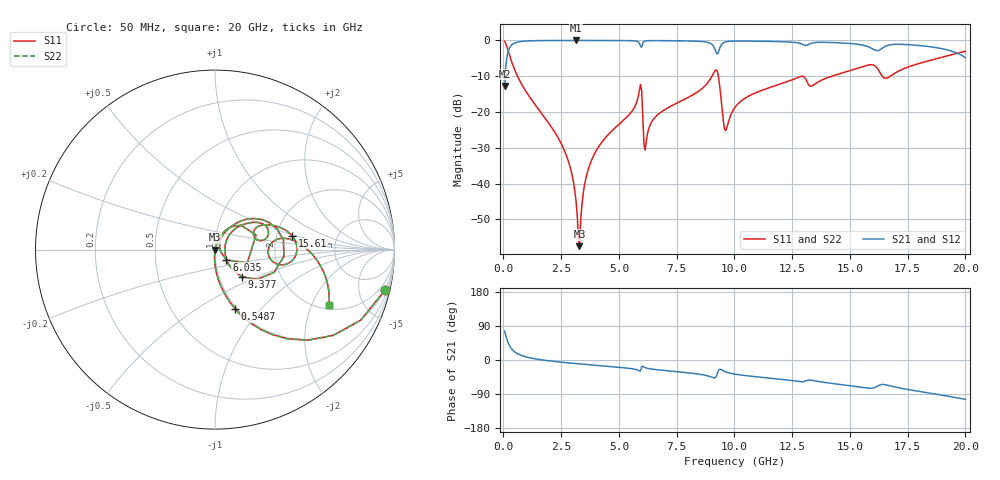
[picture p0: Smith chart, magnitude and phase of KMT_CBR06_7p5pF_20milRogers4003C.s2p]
! Data measured by Modelithics Inc. support@modelithics.com 813-866-6335
! KEMET CBR0603 7.5pF, Pad Width= 0.851mm, Pad Length= 0.64mm, Pad Gap= 0.62mm, 20mil Rogers 4003C substrate Data, January 2022
# hz S ma R 50
! 2 Port Network Data from SP1.SP block
! freq  magS11  angS11  magS21  angS21  magS12  angS12  magS22  angS22
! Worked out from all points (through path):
!   401 points, 50 MHz to 20 GHz, reference 50 ohm
!   highest |S21| = -0.01 dB at 3.142 GHz (marker M1); lowest = -12.7 dB at 50 MHz (marker M2)
!   group delay of S21, straight-line fit = 14.8 ps
!   lowest |S11| = -57.5 dB at 3.292 GHz (marker M3), VSWR 1.00, Z = 50.1 + j0.0443 ohm
!   |S11| at or under -10 dB: 610.2 MHz to 9.026 GHz (8.416 GHz wide, 175 % of centre); 9.303 GHz to 14.21 GHz (4.909 GHz wide, 41.8 % of centre); 16.4 GHz to 16.75 GHz (342.3 MHz wide, 2.07 % of centre)
!   |S22| runs from -57.5 to -0.2 dB; largest |S21 - S12| = 0
!   S11 on the Smith chart (normalised r, x): 50 MHz: 0.98, -8.32; 548.8 MHz: 0.98, -0.74; 6.035 GHz: 1.13, -0.13; 9.377 GHz: 1.28, -0.40; 15.61 GHz: 2.43, +0.47; 20 GHz: 2.21, -2.70
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5e7  0.9728 -13.5  0.2312 76.5  0.2312 76.5  0.9728 -13.5
2.495e8  0.6422 -50.8  0.7658 39.2  0.7658 39.2  0.6422 -50.8
5.4875e8  0.3494 -71.1  0.9363 18.7  0.9363 18.7  0.3494 -71.1
2.593625e9  0.03125 -94.3  0.9984 -6.3  0.9984 -6.3  0.03125 -94.3
3.14225e9  0.005735 -88.0  0.9987 -9.4  0.9987 -9.4  0.005735 -88.0
3.291875e9  0.001339 19.3  0.9987 -10.2  0.9987 -10.2  0.001339 19.3
3.391625e9  0.004876 65.2  0.9987 -10.8  0.9987 -10.8  0.004876 65.2
3.641e9  0.01463 73.0  0.9985 -12.1  0.9985 -12.1  0.01463 73.0
4.13975e9  0.03347 72.9  0.9979 -14.7  0.9979 -14.7  0.03347 72.9
5.885375e9  0.1982 43.0  0.9209 -29.1  0.9209 -29.1  0.1982 43.0
6.035e9  0.08556 -42.2  0.922 -16.5  0.922 -16.5  0.08556 -42.2
6.184625e9  0.03969 49.4  0.986 -21.2  0.986 -21.2  0.03969 49.4
6.73325e9  0.09481 61.9  0.9921 -26.2  0.9921 -26.2  0.09481 61.9
9.177125e9  0.3847 8.0  0.7257 -46.4  0.7257 -46.4  0.3847 8.0
9.376625e9  0.2122 -45.3  0.7985 -24.5  0.7985 -24.5  0.2122 -45.3
9.626e9  0.05521 6.5  0.9556 -31.5  0.9556 -31.5  0.05521 6.5
1.0025e10  0.1163 45.8  0.9791 -37.4  0.9791 -37.4  0.1163 45.8
1.2818e10  0.3099 25.8  0.9122 -57.0  0.9122 -57.0  0.3099 25.8
1.336662e10  0.2322 22.9  0.9203 -53.8  0.9203 -53.8  0.2322 22.9
1.5611e10  0.4355 10.4  0.8505 -73.0  0.8505 -73.0  0.4355 10.4
1.670825e10  0.3104 5.5  0.8651 -67.9  0.8651 -67.9  0.3104 5.5
2e10  0.7054 -25.8  0.5757 -103.8  0.5757 -103.8  0.7054 -25.8
